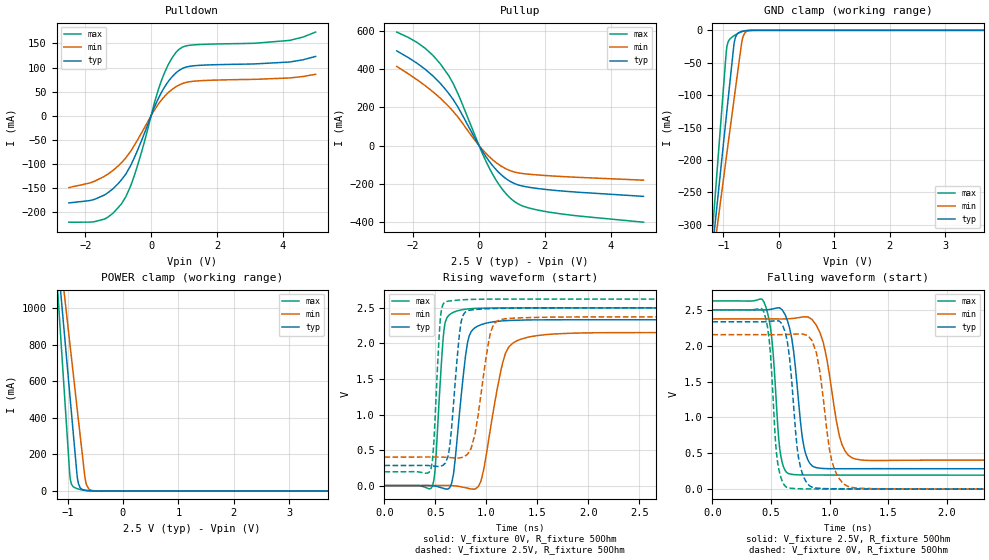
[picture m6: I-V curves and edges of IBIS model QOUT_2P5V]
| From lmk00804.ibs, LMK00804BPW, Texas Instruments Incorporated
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|   Model QOUT 2.5VCC
[Model]   QOUT_2P5V
Model_type   3-state
Polarity   Non-Inverting
Vmeas = 1.25
Vref = 2.5
Cref = 15pF
Rref = 50
|   typ   min   max
|   (fast PVT)   (slow PVT)   (nom PVT)
C_comp   0.315p   0.300p   0.317p
|C_comp (Hi state)   0.315p   0.300p   0.317p
|C_comp (Low state)   0.358p   0.325p   0.360p
[Voltage Range]   2.5   2.375   2.625
[Temperature Range]   45   125   -40
[Pullup Reference]   2.5   2.375   2.625
[Pulldown Reference]   0   -0   0
[Power Clamp Reference]   2.5   2.375   2.625
[GND Clamp Reference]   0   0   0
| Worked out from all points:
|   slope of the pulldown table from 0 to 0.375 V, typ, clamps not added: 6.74 ohm
|   slope of the pullup table from 0 to 0.375 V, typ, clamps not added: 3.87 ohm
|   GND clamp passes 1 mA (typ) near -0.63 V on its own axis
|   POWER clamp passes 1 mA (typ) near -0.60 V on its own axis
|   falling waveform, V_fixture 2.5V, R_fixture 50Ohm: 20-80 % time 85.5ps typ, 122ps min, 63ps max; typ from 2.5 V to 0.284 V
|   rising waveform, V_fixture 0V, R_fixture 50Ohm: 20-80 % time 99.2ps typ, 160ps min, 62.7ps max; typ from 0 V to 2.33 V
|   rising waveform, V_fixture 2.5V, R_fixture 50Ohm: 20-80 % time 77.5ps typ, 120ps min, 50.7ps max; typ from 0.283 V to 2.5 V
|   falling waveform, V_fixture 0V, R_fixture 50Ohm: 20-80 % time 76.9ps typ, 107ps min, 57.7ps max; typ from 2.33 V to 0 V
[Pulldown]
|   Voltage   I(typ)   I(min)   I(max)
-2.5V     -180.9mA   -149mA     -220.8mA
-1.427V   -164.7mA   -126mA     -214.6mA
-902.5mV  -133mA     -97.59mA   -182.9mA
-617.5mV  -102.8mA   -73.4mA    -144.9mA
-475mV    -81.65mA   -57.57mA   -116.8mA
117.5mV   20.26mA    13.51mA    30.79mA
327.5mV   50.02mA    33.57mA    75.23mA
537.5mV   72.43mA    48.86mA    108mA
852.5mV   94.11mA    63.82mA    138mA
1.377V    104.1mA    72.07mA    147.4mA
4.205V    111.4mA    78.31mA    156.2mA
5V        123mA      85.96mA    173.5mA
[GND Clamp]
|   Voltage   I(typ)   I(min)   I(max)
-2.5V     -1.415A    -1.22A     -1.766A
-1.195V   -334.9mA   -357.1mA   -306.7mA
-1.188V   -328.8mA   -352.2mA   -298.3mA
-1.165V   -310.3mA   -337.4mA   -273.2mA
-1V       -175.1mA   -229.9mA   -89.33mA
-940mV    -126.3mA   -191mA     -26.81mA
-910mV    -101.9mA   -171.6mA   -16.71mA
-805mV    -18.96mA   -104.1mA   -8.087mA
-707.5mV  -2.832mA   -42.12mA   -3.469mA
-647.5mV  -1.202mA   -10.08mA   -1.571mA
-512.5mV  -90.83uA   -273uA     -90.78uA
5V        0A         0A         0A
[Pullup]
|   Voltage   I(typ)   I(min)   I(max)
-2.5V     495.5mA    414.2mA    594.1mA
-1.63V    398.4mA    312.8mA    508.1mA
-1.188V   327.4mA    249.4mA    430mA
-925mV    273.4mA    205mA      367.1mA
-617.5mV  194.3mA    143.8mA    262.3mA
12.5mV    -3.731mA   -2.647mA   -5.236mA
327.5mV   -86.54mA   -61.31mA   -123mA
665mV     -151.7mA   -107mA     -219mA
1.062V    -198mA     -138.3mA   -291.7mA
1.385V    -214.6mA   -148.2mA   -320.5mA
2.112V    -231.8mA   -158.4mA   -348.5mA
5V        -266.4mA   -181.7mA   -401.8mA
[POWER Clamp]
|   Voltage   I(typ)   I(min)   I(max)
-2.5V     5.858A     5.069A     7.322A
-1.202V   1.355A     1.471A     1.206A
-1.157V   1.201A     1.347A     996.9mA
-1.09V    970.3mA    1.163A     683.1mA
-955mV    510.5mA    795.6mA    73.33mA
-902.5mV  332.4mA    653.1mA    23.19mA
-835mV    104.1mA    470.5mA    13.03mA
-805mV    40.8mA     389.5mA    10.33mA
-775mV    18.28mA    308.6mA    7.977mA
-677.5mV  3.36mA     57.37mA    2.596mA
-572.5mV  603.8uA    3.442mA    401.1uA
5V        0A         0A         0A
[Ramp]
R_load = 50
|   typ   min   max
dV/dt_r   1.40029/9.92102e-11   1.29238/1.59962e-10   1.50042/6.26596e-11
dV/dt_f   1.3299/8.55078e-11   1.18342/1.21757e-10   1.458/6.30108e-11
[Falling Waveform]
V_fixture = 2.5V
V_fixture_min = 2.375V
V_fixture_max = 2.625V
R_fixture = 50Ohm
C_fixture = 0F
|   Time   V(typ)   V(min)   V(max)
0s        2.5V       2.375V     2.625V
438.9ps   2.499V     2.375V     2.615V
507.8ps   2.511V     2.374V     2.091V
575ps     2.527V     2.374V     557mV
649.6ps   2.297V     2.377V     217.5mV
781.3ps   585.5mV    2.403V     198.2mV
870.5ps   308.3mV    2.322V     197.5mV
1.083ns   285.2mV    743.7mV    197.2mV
1.187ns   285.5mV    440.7mV    197.1mV
3.9ns     283.5mV    402.6mV    195mV
[Rising Waveform]
V_fixture = 0V
V_fixture_min = 0V
V_fixture_max = 0V
R_fixture = 50Ohm
C_fixture = 0F
|   Time   V(typ)   V(min)   V(max)
0s        435.7pV    13.72nV    389.9pV
469.8ps   -1.428mV   429uV      -5.159mV
495.5ps   -6.557mV   742.3uV    205.7mV
585.2ps   -42.07mV   1.838mV    2.21V
669.2ps   107.4mV    -1.2mV     2.434V
813.1ps   2.003V     -36.26mV   2.485V
916.8ps   2.246V     -20.12mV   2.495V
1.157ns   2.318V     1.72V      2.5V
1.292ns   2.326V     2.033V     2.5V
3.9ns     2.334V     2.154V     2.501V
[Rising Waveform]
V_fixture = 2.5V
V_fixture_min = 2.375V
V_fixture_max = 2.625V
R_fixture = 50Ohm
C_fixture = 0F
|   Time   V(typ)   V(min)   V(max)
0s        282.9mV    401.4mV    194.7mV
457ps     279mV      401.9mV    240.3mV
546.7ps   270.8mV    401.3mV    2.33V
595.7ps   315.1mV    398.9mV    2.582V
640.1ps   551.8mV    394.8mV    2.598V
751.8ps   2.303V     393.2mV    2.613V
813.1ps   2.458V     438.8mV    2.618V
1.037ns   2.49V      2.136V     2.624V
1.129ns   2.494V     2.331V     2.624V
3.9ns     2.5V       2.374V     2.625V
[Falling Waveform]
|Gnd
V_fixture = 0V
V_fixture_min = 0V
V_fixture_max = 0V
R_fixture = 50Ohm
C_fixture = 0F
|   Time   V(typ)   V(min)   V(max)
0s        2.334V     2.155V     2.501V
438.9ps   2.334V     2.154V     2.472V
484.4ps   2.34V      2.154V     2.089V
556.2ps   2.348V     2.154V     375.9mV
631.8ps   2.114V     2.157V     28.21mV
735ps     436.3mV    2.165V     6.083mV
852ps     26.69mV    2.061V     2.919mV
1.016ns   5.902mV    409.4mV    2.393mV
1.157ns   3.593mV    37.96mV    2.166mV
3.9ns     479.4uV    905.3uV    267.3uV
